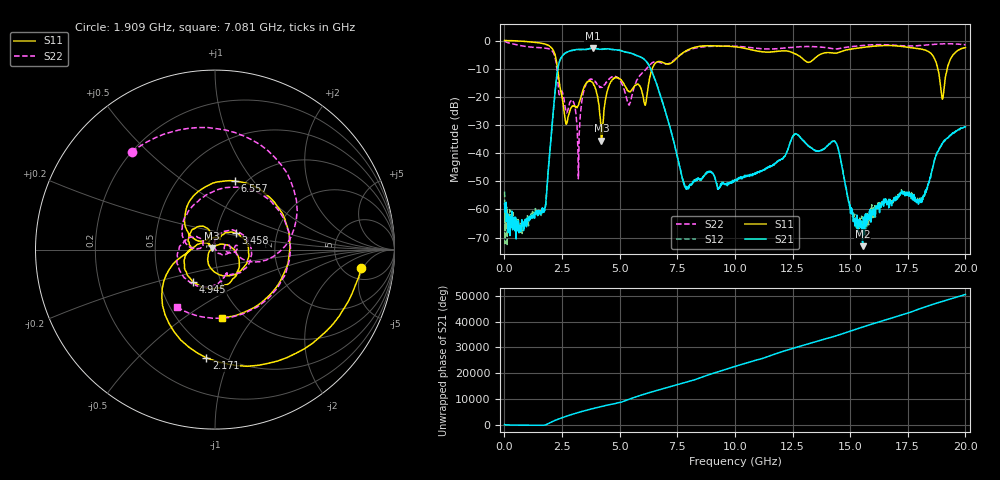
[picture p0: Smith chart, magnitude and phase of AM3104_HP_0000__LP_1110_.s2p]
!Created with skrf (http://scikit-rf.org).
# Hz S RI R 50.0
!freq ReS11 ImS11 ReS21 ImS21 ReS12 ImS12 ReS22 ImS22
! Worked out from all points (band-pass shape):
!   1601 points, 10 MHz to 20 GHz, reference 50 ohm
!   highest |S21| = -2.73 dB at 3.833 GHz (marker M1); lowest = -73.1 dB at 15.54 GHz (marker M2)
!   |S21| within 3 dB of the highest: 2.494 GHz to 5.882 GHz (3.388 GHz wide, 80.9 % of centre)
!   lowest |S11| = -35.6 dB at 4.208 GHz (marker M3), VSWR 1.03, Z = 48.5 + j0.653 ohm
!   |S11| at or under -10 dB: 2.304 GHz to 6.414 GHz (4.11 GHz wide, 94.3 % of centre); 18.8 GHz to 19.21 GHz (407.5 MHz wide, 2.14 % of centre)
!   |S22| runs from -49.1 to -0.2 dB; largest |S21 - S12| = 0.0061
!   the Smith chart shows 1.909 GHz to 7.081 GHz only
!   S11 on the Smith chart (normalised r, x): 1.909 GHz: 7.24, -4.56; 2.171 GHz: 0.43, -0.82; 3.458 GHz: 1.24, +0.23; 4.945 GHz: 0.74, -0.28; 6.557 GHz: 0.90, +0.81; 7.081 GHz: 0.80, -0.71
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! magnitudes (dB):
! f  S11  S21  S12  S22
! 10 MHz  0.0  -57.9  -53.7  -0.2
! 1.659 GHz  -1.1  -60.6  -60.4  -2.6
! 1.909 GHz  -1.7  -45.4  -45.7  -2.9
! 2.171 GHz  -4.4  -20.6  -20.6  -5.2
! 2.671 GHz  -29.6  -4.3  -4.3  -25.2
! 3.346 GHz  -19.2  -3.2  -3.2  -22.4
! 3.458 GHz  -16.5  -3.2  -3.1  -17.5
! 3.833 GHz  -15.0  -2.7  -2.7  -13.9
! 4.208 GHz  -35.6  -3.1  -3.1  -16.6
! 4.945 GHz  -13.2  -3.4  -3.4  -13.4
! 6.557 GHz  -8.0  -14.4  -14.4  -7.5
! 6.682 GHz  -7.5  -17.4  -17.4  -7.6
! 7.081 GHz  -8.3  -27.9  -28.0  -8.3
! 7.881 GHz  -3.7  -52.7  -51.8  -3.9
! 10.01 GHz  -2.2  -49.5  -49.7  -2.0
! 13.34 GHz  -7.2  -38.3  -38.2  -2.2
! 14.38 GHz  -4.5  -36.4  -36.3  -3.0
! 15.54 GHz  -2.5  -73.1  -65.7  -1.8
! 16.68 GHz  -1.8  -59.4  -56.4  -1.6
! 18.06 GHz  -3.0  -56.6  -56.7  -1.8
! 19 GHz  -20.8  -36.6  -36.6  -1.2
! 20 GHz  -2.5  -30.7  -30.6  -1.5
